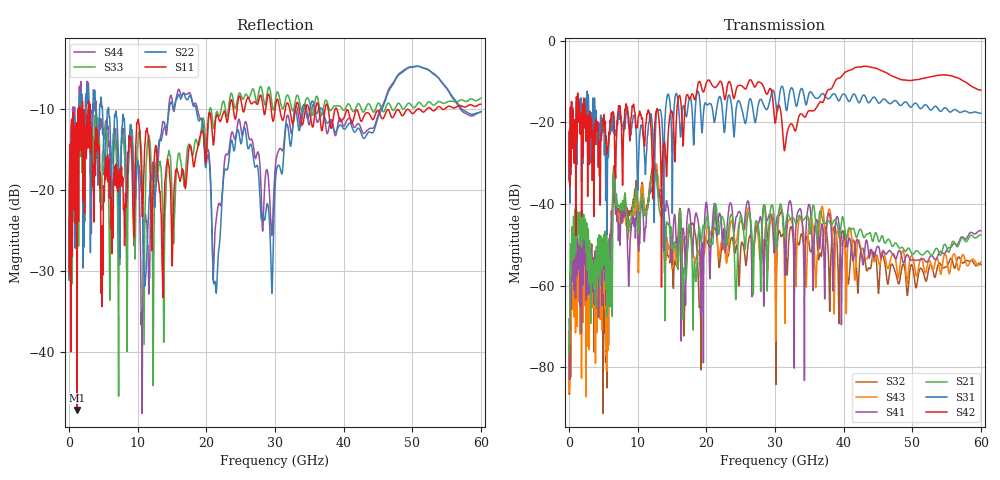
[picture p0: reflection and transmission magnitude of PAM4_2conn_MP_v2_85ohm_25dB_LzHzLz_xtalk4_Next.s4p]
! Info: Touchstone file created by Circ.  Input file=FAB50GbE_2conn_Midplane_Examax_Topo2_v2_85ohm_25dB_LzHzLz.circ
# Hz S RI R 50
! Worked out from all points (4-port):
!   6000 points, 10 MHz to 60 GHz, reference 50 ohm
!   strongest paths, dB at 10 MHz, 15.01 GHz, 30.01 GHz, 45.01 GHz, 60 GHz:
!     S42: -34.0, -17.4, -20.2, -7.0, -12.1
!     S31: -34.6, -32.6, -13.8, -15.1, -17.8
!     S21: -75.9, -51.0, -47.3, -48.7, -47.6
!     S41: -68.1, -54.9, -48.7, -50.4, -46.6
!     S43: -71.3, -55.9, -55.6, -53.5, -54.3
!     S32: -75.1, -54.2, -52.4, -60.5, -54.9
!   lowest |S11| = -47.2 dB at 1.17 GHz (marker M1), VSWR 1.01, Z = 49.6 + j0.235 ohm
!   |S11| at or under -10 dB: start of sweep to 1.468 GHz; 3.069 GHz to 23.34 GHz (20.27 GHz wide, 154 % of centre); 39.04 GHz to 49.25 GHz (10.21 GHz wide, 23.1 % of centre)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
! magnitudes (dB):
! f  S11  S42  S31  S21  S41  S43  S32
! 10 MHz  -30.3  -34.0  -34.6  -75.9  -68.1  -71.3  -75.1
! 1.17 GHz  -47.2  -24.3  -30.3  -48.1  -53.1  -57.6  -54.9
! 12.64 GHz  -14.4  -17.7  -20.1  -32.3  -31.7  -30.2  -30.3
! 19.09 GHz  -13.3  -10.2  -15.4  -46.9  -53.8  -54.3  -65.1
! 21.27 GHz  -12.0  -11.5  -19.4  -40.5  -40.4  -42.4  -46.1
! 28.45 GHz  -10.6  -11.8  -16.2  -40.4  -53.7  -48.8  -40.2
! 60 GHz  -9.4  -12.1  -17.8  -47.6  -46.6  -54.3  -54.9
